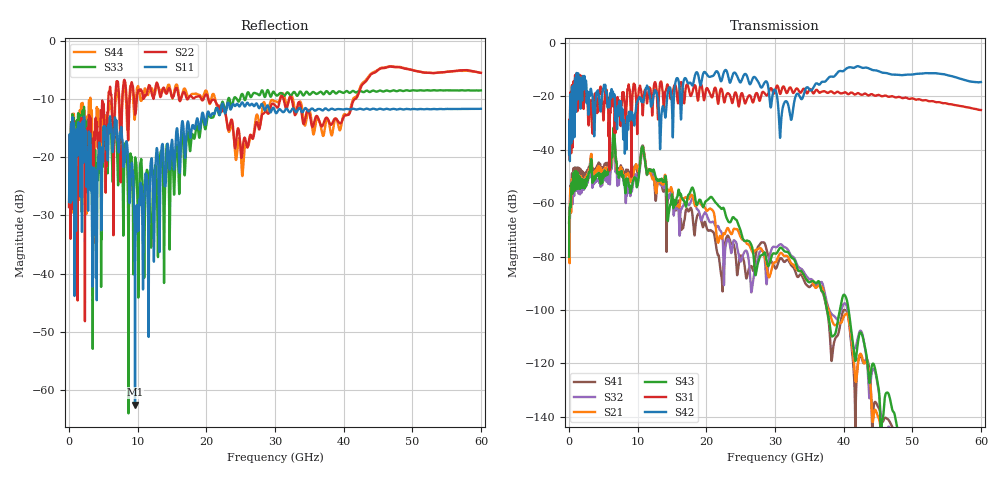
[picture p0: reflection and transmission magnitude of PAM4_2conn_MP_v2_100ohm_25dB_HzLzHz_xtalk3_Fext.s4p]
! Info: Touchstone file created by Circ.  Input file=FAB50GbE_2conn_Midplane_Examax_Topo2_v2_100ohm_25dB_HzLzHz.circ
# Hz S RI R 50
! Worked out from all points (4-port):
!   6000 points, 10 MHz to 60 GHz, reference 50 ohm
!   strongest paths, dB at 10 MHz, 15.01 GHz, 30.01 GHz, 45.01 GHz, 60 GHz:
!     S42: -41.6, -24.7, -17.5, -10.5, -14.7
!     S31: -41.0, -18.8, -17.9, -19.4, -25.1
!     S43: -80.0, -56.8, -78.9, -127.9, -176.6
!     S21: -63.9, -55.1, -82.2, -140.0, -183.7
!     S32: -67.7, -55.6, -76.4, -128.8, -181.1
!     S41: -67.1, -56.2, -84.3, -136.2, -191.8
!   lowest |S11| = -62.5 dB at 9.61 GHz (marker M1), VSWR 1.00, Z = 50.1 - j0.0174 ohm
!   |S11| at or under -10 dB: start of sweep to end of sweep
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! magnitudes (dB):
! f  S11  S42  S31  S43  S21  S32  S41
! 10 MHz  -27.7  -41.6  -41.0  -80.0  -63.9  -67.7  -67.1
! 640 MHz  -16.7  -16.1  -14.6  -50.1  -49.4  -52.0  -47.0
! 6.45 GHz  -17.5  -19.6  -23.8  -32.6  -35.5  -37.5  -33.2
! 9.61 GHz  -62.5  -26.8  -16.1  -50.7  -46.6  -49.6  -46.1
! 22.1 GHz  -12.0  -14.3  -17.2  -61.9  -72.5  -70.4  -85.8
! 30.8 GHz  -11.9  -33.6  -19.0  -76.7  -78.7  -75.4  -80.6
! 60 GHz  -11.7  -14.7  -25.1  -176.6  -183.7  -181.1  -191.8
